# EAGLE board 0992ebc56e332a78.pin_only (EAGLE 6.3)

Size 12.7 x 10.16 mm. Coordinates in mm from the lower left corner, seen from the top.
Outline: 2.54,10.16 10.16,10.16 arc-90 12.7,7.62 12.7,2.54 arc-90 10.16,0 2.54,0 arc-90 0,2.54 0,7.62 arc-90 2.54,10.16
Copper layers (1*16): Top 0.035mm / dielectric 1.5mm / Bottom 0.035mm
Design rules "default": minimum track width 10mil, minimum drill 19mil, track to track 8mil, track to pad 8mil, pad to pad 8mil, via to via 8mil, smd to smd 8mil, copper to edge 10mil, drill to drill 8mil, minimum pad ring 10mil, minimum via ring 8mil, stop-mask expansion 4mil, vias tented up to drill 20mil, thermal gap 10mil
Holes 2.2 mm at 6.35,8.89 6.35,1.27

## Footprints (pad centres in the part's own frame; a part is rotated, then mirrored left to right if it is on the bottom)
C0603K = smd 1.05 x 1.08: 1 -0.875,0; 2 0.875,0
1X03-CLEANBIG = drill 1.016 pad 1.676: 1 -2.54,0; 2 0,0; 3 2.54,0
WS28115050 = smd 2 x 1.1: DI 2,0; DO 2,-1.7; LEDVDD -2,0; NC -2,1.7; VDD 2,1.7; VSS -2,-1.7
R0603 = smd 1 x 1.1: 1 -0.85,0; 2 0.85,0

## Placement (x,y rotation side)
C1  1uF  [C0603K]  9.27,9.02 0 top
JP1  [1X03-CLEANBIG]  1.27,5.08 90 top
JP2  [1X03-CLEANBIG]  11.43,5.08 270 top
LED1  WS28115050  [WS28115050]  6.35,5.08 0 top
R1  1.0K  [R0603]  3.43,9.02 180 top
R2  22  [R0603]  9.27,1.14 0 top
R3  22  [R0603]  3.43,1.14 180 top
U$1  [ADAFRUIT_2.5MM]  10.03,6.73 0 bottom

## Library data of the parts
C1 JP1 JP2 R1-R3 = adafruit
LED1 U$1 = microbuilder

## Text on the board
bPlace: v1 | NeoPixel | V+ 5-9V
tDocu: + | + | G | G | In | O

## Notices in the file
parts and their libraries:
microbuilder: This work is placed in the public domain, and may be freely used for commercial and non-commercial work with the following conditions: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
